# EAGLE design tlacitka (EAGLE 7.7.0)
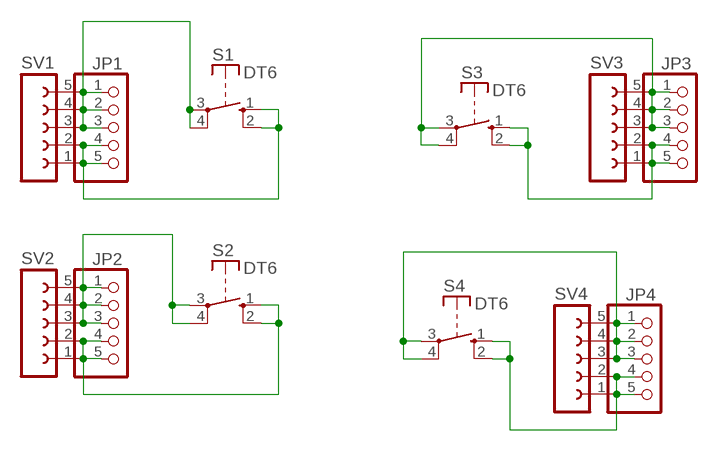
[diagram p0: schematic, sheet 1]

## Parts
JP1  PINHD-1X5  [1X05]
JP2  PINHD-1X5  [1X05]
JP3  PINHD-1X5  [1X05]
JP4  PINHD-1X5  [1X05]
S1  DT6  [DT6]
S2  DT6  [DT6]
S3  DT6  [DT6]
S4  DT6  [DT6]
SV1  FE05-1  [FE05-1]
SV2  FE05-1  [FE05-1]
SV3  FE05-1  [FE05-1]
SV4  FE05-1  [FE05-1]

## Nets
N$1: JP1.4 JP1.5 S1.1(S) S1.2(S) SV1.1 SV1.2
N$2: JP4.4 JP4.5 S4.1(S) S4.2(S) SV4.1 SV4.2
N$3: JP1.1 JP1.2 JP1.3 S1.3(P) S1.4(P) SV1.3 SV1.4 SV1.5
N$6: JP2.1 JP2.2 JP2.3 S2.3(P) S2.4(P) SV2.3 SV2.4 SV2.5
N$9: JP2.4 JP2.5 S2.1(S) S2.2(S) SV2.1 SV2.2
N$11: JP3.1 JP3.2 JP3.3 S3.3(P) S3.4(P) SV3.3 SV3.4 SV3.5
N$14: JP3.4 JP3.5 S3.1(S) S3.2(S) SV3.1 SV3.2
N$18: JP4.1 JP4.2 JP4.3 S4.3(P) S4.4(P) SV4.3 SV4.4 SV4.5

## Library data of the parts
JP1-JP4 = pinhead:PINHD-1X5: PIN HEADER
S1-S4 = switch-misc:DT: ITT SWITCH
SV1-SV4 = con-lsta:FE05-1: FEMALE HEADER; OC_FARNELL: unknown; OC_NEWARK: unknown

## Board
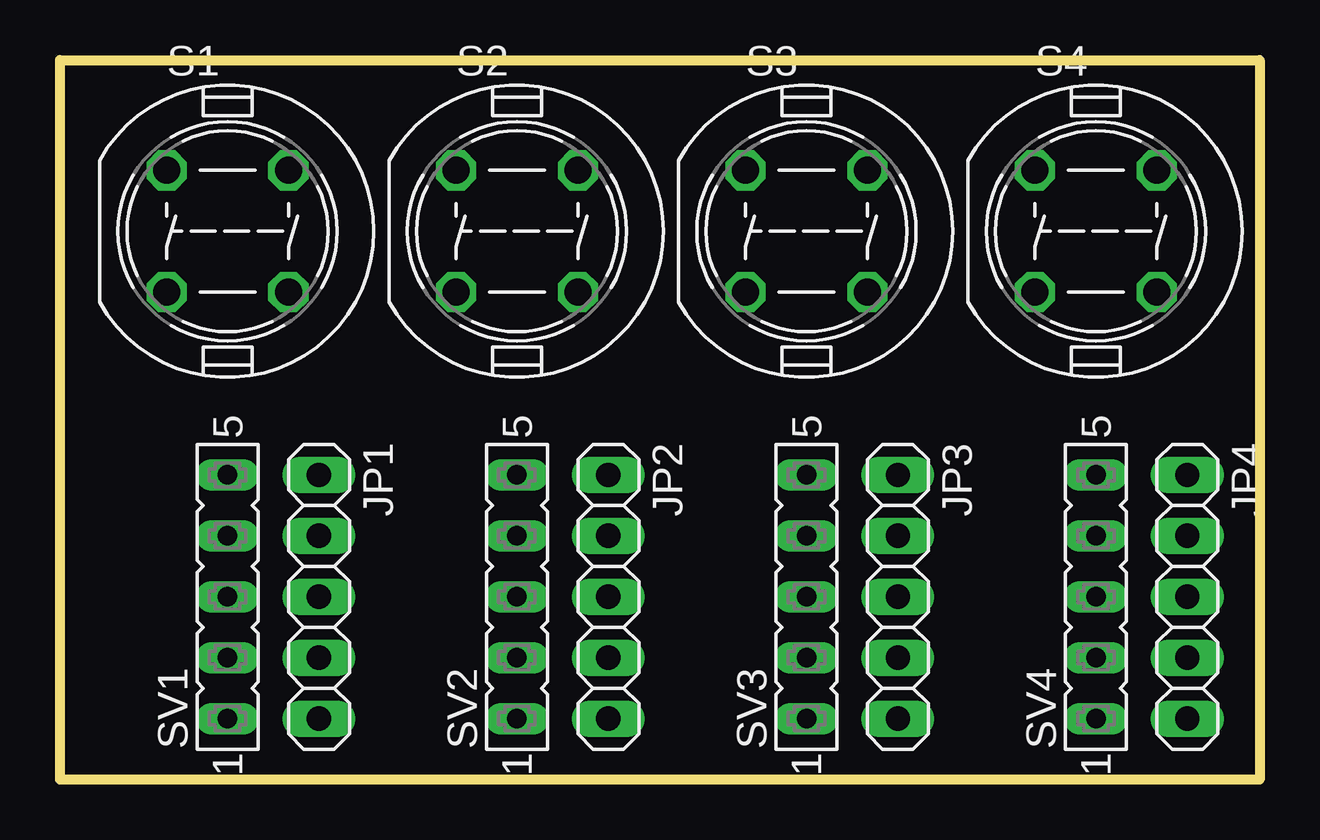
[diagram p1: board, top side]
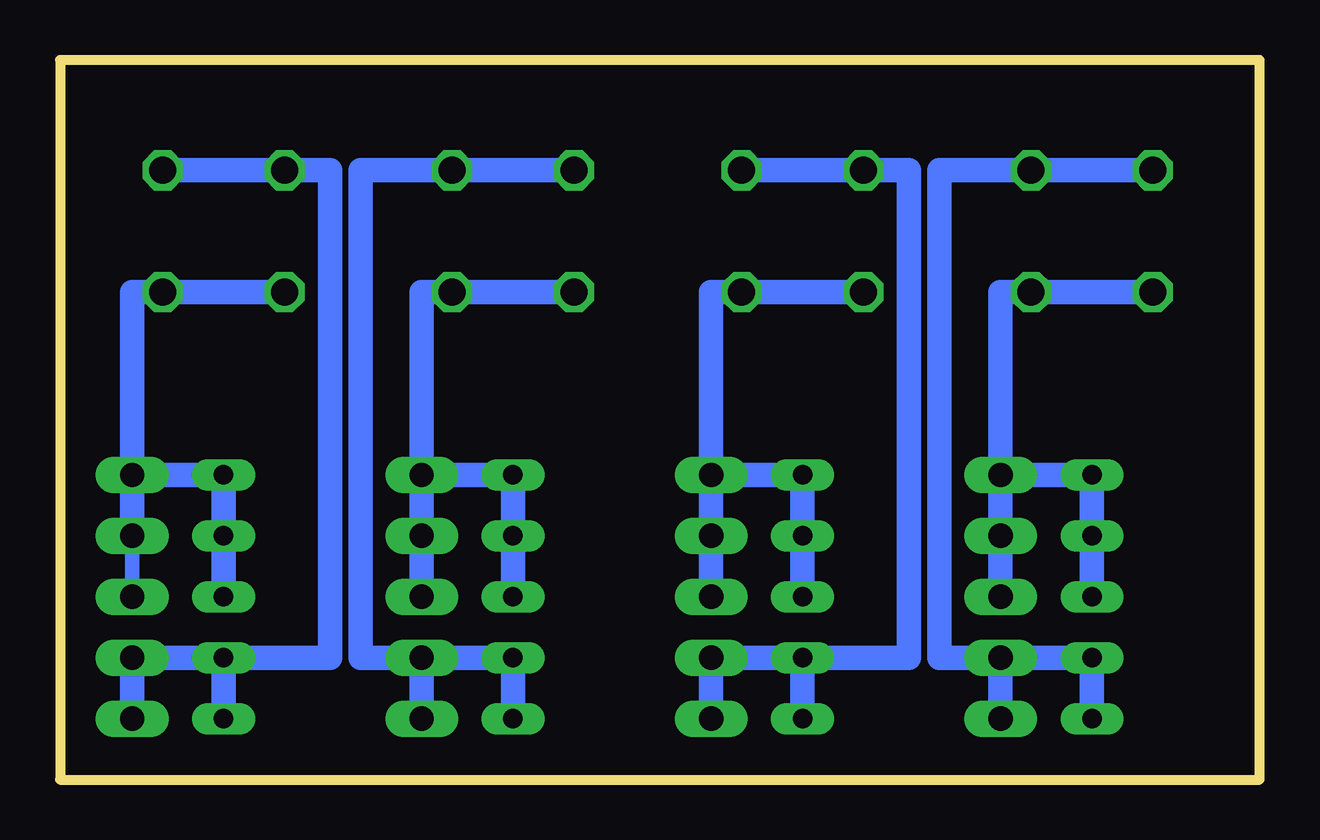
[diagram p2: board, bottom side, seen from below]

Size 50 x 30 mm. Coordinates in mm from the lower left corner, seen from the top.
Outline: 0,0 0,30 50,30 50,0 0,0
Copper layers (1*16): Top 0.035mm / dielectric 1.5mm / Bottom 0.035mm
Design rules "default": minimum track width 10mil, minimum drill 24mil, track to track 8mil, track to pad 8mil, pad to pad 8mil, via to via 8mil, smd to smd 8mil, copper to edge 40mil, drill to drill 8mil, minimum pad ring 10mil, minimum via ring 8mil, stop-mask expansion 4mil, vias tented up to drill 0mil, thermal gap 10mil

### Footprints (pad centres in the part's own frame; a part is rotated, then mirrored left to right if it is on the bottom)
1X05 = drill 1.016 long: 1 -5.08,0; 2 -2.54,0; 3 0,0; 4 2.54,0; 5 5.08,0
DT6 = drill 1.118 octagon: 1 -2.54,2.54; 2 2.54,2.54; 3 2.54,-2.54; 4 -2.54,-2.54
FE05-1 = drill 0.813 long: 1 -5.08,0; 2 -2.54,0; 3 0,0; 4 2.54,0; 5 5.08,0

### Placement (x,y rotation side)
JP1  10.79,7.62 270 top
JP2  22.86,7.62 270 top
JP3  34.92,7.62 270 top
JP4  46.99,7.62 270 top
S1  6.99,22.86 0 top
S2  19.05,22.86 0 top
S3  31.11,22.86 0 top
S4  43.18,22.86 0 top
SV1  6.99,7.62 90 top
SV2  19.05,7.62 90 top
SV3  31.11,7.62 90 top
SV4  43.18,7.62 90 top

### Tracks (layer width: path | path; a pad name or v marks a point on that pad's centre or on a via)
N$1
  Bottom 1.016: S1.1 S1.2 13.34,25.4 13.34,5.08 JP1.4 | SV1.1 SV1.2 JP1.4 | JP1.4 JP1.5
N$2
  Bottom 0.61: S4.1 S4.2
  Bottom 1.016: SV4.1 SV4.2 | SV4.2 JP4.4 JP4.5 | S4.2 38.73,25.4 38.73,5.08 SV4.2
N$3
  Bottom 1.016: S1.4 S1.3 10.79,20.32 JP1.1 | SV1.3 SV1.4 SV1.5 JP1.1 | JP1.3 JP1.2 JP1.1
N$6
  Bottom 1.016: S2.4 S2.3 22.86,20.32 JP2.1 | SV2.3 SV2.4 SV2.5 JP2.1 | JP2.1 JP2.2 JP2.3
N$9
  Bottom 1.016: S2.2 S2.1 14.61,25.4 14.61,5.08 JP2.4 | SV2.1 SV2.2 JP2.4 | JP2.5 JP2.4
N$11
  Bottom 1.016: S3.4 S3.3 34.92,20.32 JP3.1 | JP3.3 JP3.2 JP3.1 | JP3.1 SV3.5 SV3.4 SV3.3
N$14
  Bottom 1.016: S3.1 S3.2 37.47,25.4 37.47,5.08 JP3.4 | SV3.1 SV3.2 JP3.4 | JP3.4 JP3.5
N$18
  Bottom 0.61: JP4.2 JP4.3
  Bottom 1.016: S4.4 S4.3 46.99,20.32 JP4.1 | SV4.3 SV4.4 SV4.5 JP4.1 | JP4.1 JP4.2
